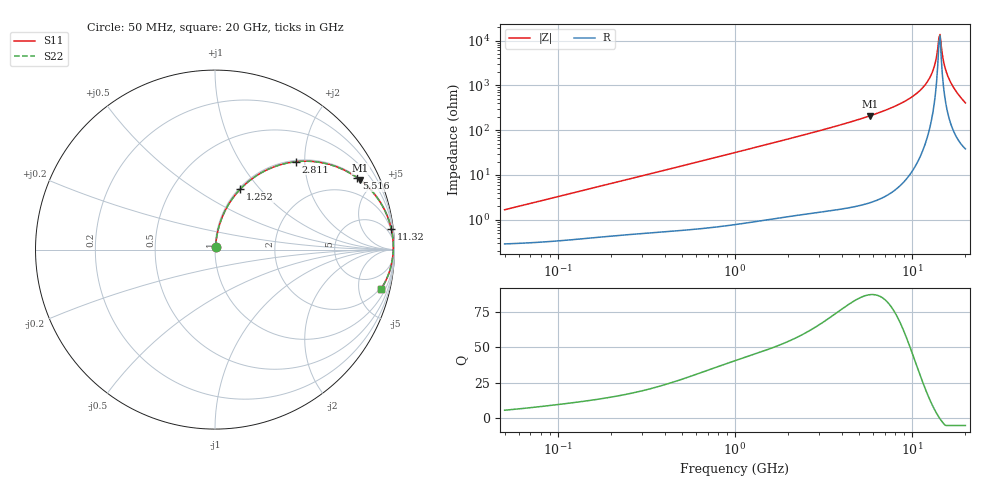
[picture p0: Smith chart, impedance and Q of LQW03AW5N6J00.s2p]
!Murata Part Number: LQW03AW5N6J00
!These Parameters are Measured in Series Mode Connection
!  o--[Z]--o
!Port1  Port2
!  o-------o
!Freq. Start=50[MHz] Stop=20[GHz], 401[Steps]
# Hz S RI R 50
!Freq.(Hz) S11(Real) S11(Imag) S21(Real) S21(Imag) S12(Real) S12(Imag) S22(Real) S22(Imag)
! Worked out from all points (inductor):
!   401 points, 50 MHz to 20 GHz, reference 50 ohm
!   read as one part in series: L = 5.26 nH near 51.52 MHz
!   highest Q = 86.8 at 5.769 GHz (marker M1), where L = 5.75 nH
!   self-resonance near 14.17 GHz
!   S11 on the Smith chart (normalised r, x): 50 MHz: 1.01, +0.03; 1.252 GHz: 1.02, +0.79; 2.811 GHz: 1.03, +1.82; 5.516 GHz: 1.05, +3.93; 11.32 GHz: 2, +17; 20 GHz: 1.77, -8.09
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5e7  0.00317 0.0164  0.9968 -0.0164  0.9968 -0.0164  0.00317 0.0164
1.364002e8  0.00571 0.0441  0.9943 -0.0441  0.9943 -0.0441  0.00571 0.0441
3.721004e8  0.019 0.116  0.981 -0.116  0.981 -0.116  0.019 0.116
1e9  0.0972 0.2842  0.9028 -0.2842  0.9028 -0.2842  0.0972 0.2842
1.251922e9  0.1418 0.3379  0.8582 -0.3379  0.8582 -0.3379  0.1418 0.3379
2.728004e9  0.4375 0.4882  0.5625 -0.4882  0.5625 -0.4882  0.4375 0.4882
2.810964e9  0.4529 0.49  0.5471 -0.49  0.5471 -0.49  0.4529 0.49
5.515528e9  0.7917 0.4003  0.2083 -0.4003  0.2083 -0.4003  0.7917 0.4003
5.769027e9  0.8102 0.3864  0.1898 -0.3864  0.1898 -0.3864  0.8102 0.3864
7.442007e9  0.8985 0.2958  0.1015 -0.2958  0.1015 -0.2958  0.8985 0.2958
9.457416e9  0.9554 0.1974  0.0446 -0.1974  0.0446 -0.1974  0.9554 0.1974
1.131968e10  0.9817 0.1171  0.0183 -0.1171  0.0183 -0.1171  0.9817 0.1171
1.220001e10  0.9884 0.0816  0.0116 -0.0816  0.0116 -0.0816  0.9884 0.0816
1.295331e10  0.9919 0.0521  0.00813 -0.0521  0.00813 -0.0521  0.9919 0.0521
1.354865e10  0.9932 0.0293  0.00679 -0.0293  0.00679 -0.0293  0.9932 0.0293
1.396067e10  0.9935 0.0136  0.00653 -0.0136  0.00653 -0.0136  0.9935 0.0136
1.438523e10  0.9932 -0.00249  0.00684 0.00249  0.00684 0.00249  0.9932 -0.00249
1.460232e10  0.9928 -0.0107  0.00722 0.0107  0.00722 0.0107  0.9928 -0.0107
1.550395e10  0.9896 -0.0447  0.0104 0.0447  0.0104 0.0447  0.9896 -0.0447
1.621653e10  0.9851 -0.0716  0.0149 0.0716  0.0149 0.0716  0.9851 -0.0716
1.774144e10  0.9691 -0.1302  0.0309 0.1302  0.0309 0.1302  0.9691 -0.1302
2e10  0.9242 -0.2214  0.0758 0.2214  0.0758 0.2214  0.9242 -0.2214
